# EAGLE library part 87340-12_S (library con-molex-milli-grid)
RECEPTACAL
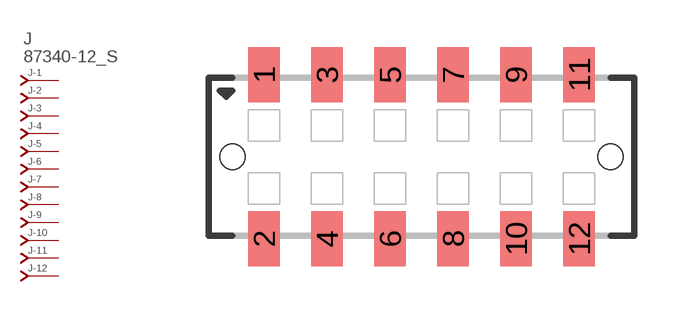
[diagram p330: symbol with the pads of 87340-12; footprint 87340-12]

Designator prefix J; gates -1=J-NV -2=J-N -3=J-N -4=J-N -5=J-N -6=J-N -7=J-N -8=J-N -9=J-N -10=J-N -11=J-N -12=J-N

## 87340-12_S  [87340-12]
1  -1:J  pas
2  -2:J  pas
3  -3:J  pas
4  -4:J  pas
5  -5:J  pas
6  -6:J  pas
7  -7:J  pas
8  -8:J  pas
9  -9:J  pas
10  -10:J  pas
11  -11:J  pas
12  -12:J  pas

## Footprint 87340-12 (pad centres in mm)
RECEPTACAL SMD Dual Row, Vertical, Low Profile
smd 1 x 1.75: 1 -5,2.6; 2 -5,-2.6; 3 -3,2.6; 4 -3,-2.6; 5 -1,2.6; 6 -1,-2.6; 7 1,2.6; 8 1,-2.6; 9 3,2.6; 10 3,-2.6; 11 5,2.6; 12 5,-2.6
hole 0.8 at -6,0
hole 0.8 at 6,0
